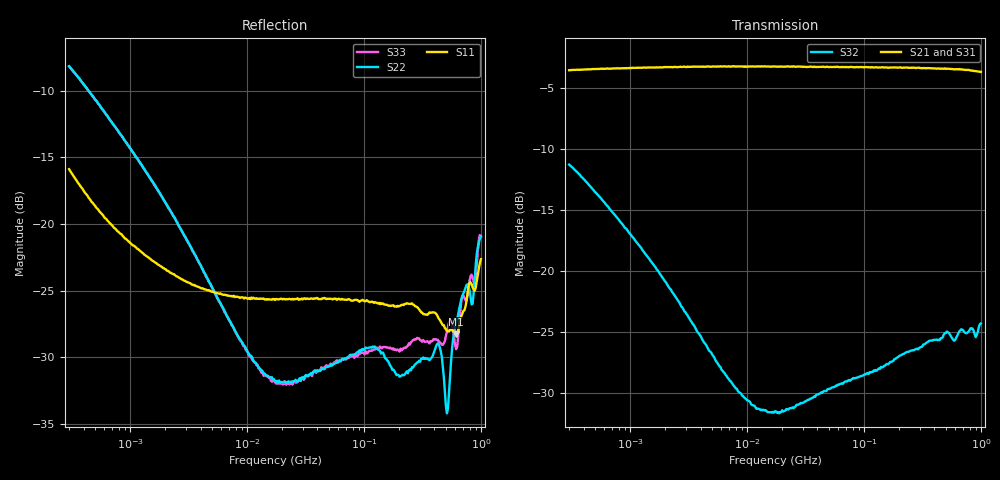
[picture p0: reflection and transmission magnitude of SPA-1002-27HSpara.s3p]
! RFMD Splitter
! SPA-1002-27H Tested 1/12/2010
! S3P Data File Format
! All S Parameters Mag in dB and Angle in Degree format
! Test Conditions: Input Power = -10dBm @ Temperature +25 deg C
! 801 Frequency points - Log Sweep
! Port 1 is Pin 1, Port 2 is Pin 3 and Port 3 is Pin 4.
! FrequencMag(S11)Angle(S1Mag(S12)Angle(S1Mag(S13)!!!!Angle(S1Mag(S14)Angle(S14)
!  Mag(S21)Angle(S2Mag(S22)Angle(S2Mag(S23)!Angle(S2Mag(S24)Angle(S24)
!  Mag(S31)Angle(S3Mag(S32)Angle(S3Mag(S33)Angle(S3Mag(S34)Angle(S34)
# Hz S  dB  R 75
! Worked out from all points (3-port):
!   401 points, 300 kHz to 1 GHz, reference 75 ohm
!   strongest paths, dB at 300 kHz, 2.28 MHz, 17.32 MHz, 131.6 MHz, 1 GHz:
!     S21: -3.6, -3.3, -3.2, -3.3, -3.7
!     S31: -3.6, -3.3, -3.3, -3.3, -3.7
!     S32: -11.3, -21.7, -31.5, -28.1, -24.3
!   lowest |S11| = -28.3 dB at 614.6 MHz (marker M1), VSWR 1.08, Z = 70.8 - j3.79 ohm
!   |S11| at or under -10 dB: start of sweep to end of sweep
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300000  -15.90 -53.1  -3.56 -172.0  -3.56 -172.1
        -3.55 -172.1  -8.17 -43.9  -11.28 150.6
        -3.56 -172.0  -11.29 150.5  -8.18 -43.9
2144961  -23.57 -25.7  -3.31 -178.5  -3.30 -178.5
         -3.29 -178.5  -18.87 -59.2  -21.35 127.9
         -3.30 -178.6  -21.37 128.2  -18.85 -59.6
1.732051e7  -25.71 -7.7  -3.26 178.9  -3.26 178.9
            -3.25 179.0  -31.79 -27.3  -31.54 171.5
            -3.25 178.9  -31.52 171.5  -31.86 -29.7
1.238394e8  -25.88 -24.7  -3.32 172.1  -3.32 171.9
            -3.32 171.9  -29.20 -31.7  -28.15 -160.3
            -3.33 171.9  -28.23 -160.2  -29.43 -39.2
2.098195e8  -26.07 -40.9  -3.34 166.8  -3.36 166.4
            -3.35 166.7  -31.38 -64.5  -26.91 -154.9
            -3.36 166.5  -26.90 -155.2  -29.49 -66.4
4.266755e8  -26.93 -90.4  -3.37 153.1  -3.44 152.7
            -3.41 153.1  -28.97 -126.8  -25.69 -148.4
            -3.43 152.7  -25.69 -148.5  -28.69 -120.8
5.121091e8  -28.04 -111.9  -3.43 147.6  -3.49 147.3
            -3.43 147.5  -34.22 -153.8  -25.06 -144.9
            -3.47 147.4  -24.98 -145.0  -28.09 -147.4
6.146491e8  -28.29 -136.2  -3.47 140.9  -3.53 140.7
            -3.47 140.7  -27.37 166.4  -25.48 -141.6
            -3.53 140.7  -25.49 -142.2  -29.40 -163.6
8.502417e8  -24.78 158.0  -3.59 124.6  -3.66 124.8
            -3.59 124.6  -25.98 129.0  -24.74 -127.1
            -3.65 124.8  -24.74 -127.0  -24.03 148.3
1e9  -22.65 119.6  -3.74 113.3  -3.78 113.9
     -3.69 113.0  -20.93 112.1  -24.33 -118.9
     -3.75 113.6  -24.32 -119.1  -20.96 129.1
